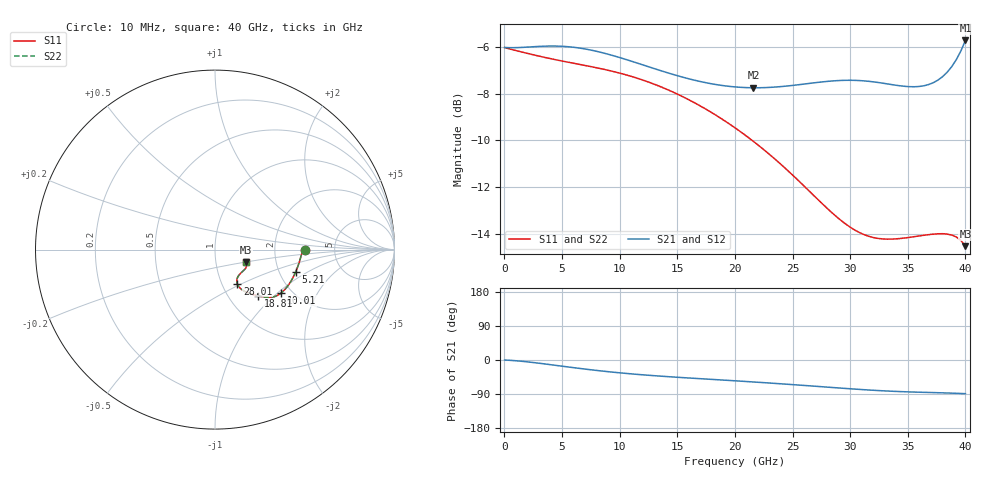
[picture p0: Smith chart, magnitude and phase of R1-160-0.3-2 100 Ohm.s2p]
!version-1
!date-09.2020
# MHz S RI R 50
!Freq ReS11 ImS11 ReS21 ImS21 ReS12 ImS12 ReS22 ImS22
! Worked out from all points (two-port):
!   101 points, 10 MHz to 40 GHz, reference 50 ohm
!   highest |S21| = -5.72 dB at 40 GHz (marker M1); lowest = -7.7 dB at 21.61 GHz (marker M2)
!   |S21| within 3 dB of the highest: start of sweep to end of sweep
!   lowest |S11| = -14.5 dB at 40 GHz (marker M3), VSWR 1.46, Z = 70.3 - j10 ohm
!   |S11| at or under -10 dB: 21.49 GHz to end of sweep
!   |S22| runs from -14.5 to -6.0 dB; largest |S21 - S12| = 0
!   S11 on the Smith chart (normalised r, x): 10 MHz: 3.00, +0.00; 5.21 GHz: 2.47, -0.77; 10.01 GHz: 1.76, -1.06; 18.81 GHz: 1.36, -0.80; 28.01 GHz: 1.18, -0.47; 40 GHz: 1.41, -0.20
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10  0.4999 0.000146  0.5 -0.000126  0.5 -0.000126  0.4999 0.000146
810  0.4938 0.0035  0.4994 -0.0136  0.4994 -0.0136  0.4938 0.0035
2010  0.4854 -0.0151  0.4991 -0.0437  0.4991 -0.0437  0.4854 -0.0151
5210  0.4502 -0.1227  0.4803 -0.1483  0.4803 -0.1483  0.4502 -0.1227
6810  0.4239 -0.175  0.4567 -0.1968  0.4567 -0.1968  0.4239 -0.175
8410  0.3955 -0.2151  0.427 -0.236  0.427 -0.236  0.3955 -0.2151
10010  0.3682 -0.242  0.395 -0.2651  0.395 -0.2651  0.3682 -0.242
11610  0.3432 -0.2574  0.3636 -0.2856  0.3636 -0.2856  0.3432 -0.2574
13610  0.3147 -0.2652  0.3274 -0.3024  0.3274 -0.3024  0.3147 -0.2652
18810  0.2404 -0.2574  0.2516 -0.3299  0.2516 -0.3299  0.2404 -0.2574
20010  0.2217 -0.2531  0.2367 -0.3369  0.2367 -0.3369  0.2217 -0.2531
21610  0.1965 -0.2458  0.2173 -0.3477  0.2173 -0.3477  0.1965 -0.2458
24410  0.1554 -0.2269  0.1831 -0.3705  0.1831 -0.3705  0.1554 -0.2269
26810  0.1304 -0.2032  0.1511 -0.3918  0.1511 -0.3918  0.1304 -0.2032
28010  0.1237 -0.1894  0.1337 -0.4014  0.1337 -0.4014  0.1237 -0.1894
30810  0.125 -0.1571  0.0912 -0.4149  0.0912 -0.4149  0.125 -0.1571
33610  0.1428 -0.1319  0.055 -0.4128  0.055 -0.4128  0.1428 -0.1319
36010  0.1603 -0.1154  0.0359 -0.4111  0.0359 -0.4111  0.1603 -0.1154
37610  0.1702 -0.1042  0.0273 -0.4248  0.0273 -0.4248  0.1702 -0.1042
38810  0.1754 -0.0926  0.0201 -0.4544  0.0201 -0.4544  0.1754 -0.0926
39610  0.1761 -0.0792  0.0139 -0.4914  0.0139 -0.4914  0.1761 -0.0792
40000  0.1747 -0.0688  0.0104 -0.5176  0.0104 -0.5176  0.1747 -0.0688
